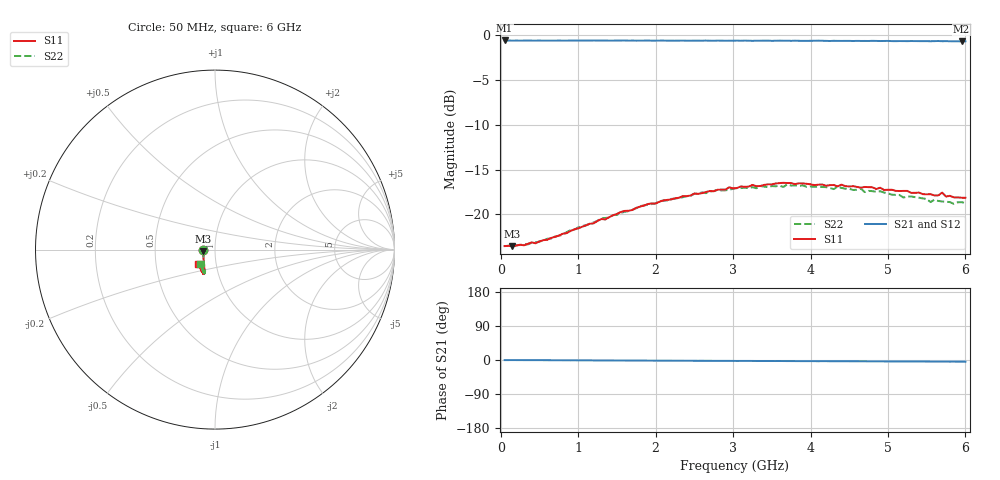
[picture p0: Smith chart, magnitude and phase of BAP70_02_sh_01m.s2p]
!	Created	by	janssen	on	Thu	Dec	12	13:21:33	MET	2002
#	HZ	S	MA	R	50
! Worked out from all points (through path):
!   120 points, 50 MHz to 6 GHz, reference 50 ohm
!   highest |S21| = -0.58 dB at 50 MHz (marker M1); lowest = -0.7 dB at 5.95 GHz (marker M2)
!   lowest |S11| = -23.6 dB at 150 MHz (marker M3), VSWR 1.14, Z = 43.8 - j0.763 ohm
!   |S11| at or under -10 dB: start of sweep to end of sweep
!   |S22| runs from -23.6 to -16.7 dB; largest |S21 - S12| = 0.0059
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5e7  0.06651 -176.3  0.9349 -0.3  0.9335 -0.4  0.06642 -176.0
1.5e8  0.06642 -172.5  0.933 -0.2  0.9323 -0.3  0.06765 -172.9
6.5e8  0.07377 -151.4  0.9333 -0.6  0.9328 -0.6  0.07322 -151.4
1.05e9  0.0852 -138.3  0.9337 -0.9  0.9331 -0.9  0.08595 -137.3
1.55e9  0.103 -127.4  0.9338 -1.3  0.932 -1.4  0.1017 -127.2
2.05e9  0.1176 -120.6  0.9332 -1.7  0.9325 -1.8  0.1185 -120.4
2.95e9  0.1416 -114.9  0.9318 -2.4  0.9318 -2.4  0.1371 -114.8
3.05e9  0.1403 -114.8  0.9331 -2.5  0.9312 -2.6  0.1401 -113.7
3.65e9  0.15 -114.6  0.9316 -2.7  0.9283 -2.9  0.1422 -114.0
3.7e9  0.1495 -115.4  0.9317 -2.8  0.9306 -2.9  0.1469 -113.8
4.05e9  0.1456 -116.7  0.9312 -3.1  0.9284 -3.1  0.1424 -115.5
4.65e9  0.1408 -120.6  0.9288 -3.5  0.9275 -3.6  0.1392 -118.5
4.7e9  0.1422 -121.4  0.929 -3.5  0.9253 -3.7  0.1331 -119.0
4.9e9  0.1408 -122.5  0.928 -3.7  0.9269 -3.8  0.1345 -120.9
5.05e9  0.1372 -124.2  0.9272 -3.8  0.9248 -3.8  0.1288 -121.4
5.5e9  0.1293 -129.1  0.9266 -4.1  0.9234 -4.2  0.1218 -127.7
5.55e9  0.1296 -129.7  0.9256 -4.1  0.9232 -4.2  0.117 -128.0
5.6e9  0.1276 -130.7  0.9267 -4.2  0.9237 -4.2  0.1207 -128.1
5.7e9  0.1322 -133.3  0.9258 -4.2  0.9229 -4.4  0.1179 -129.7
5.75e9  0.1256 -133.8  0.927 -4.3  0.9215 -4.3  0.1176 -132.0
5.95e9  0.1238 -136.2  0.9242 -4.5  0.9214 -4.5  0.117 -133.5
6e9  0.1237 -138.3  0.9251 -4.5  0.9216 -4.5  0.1155 -135.7
